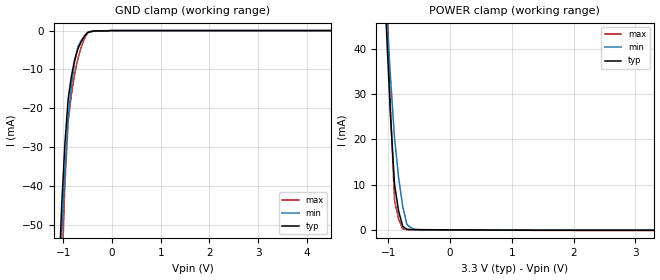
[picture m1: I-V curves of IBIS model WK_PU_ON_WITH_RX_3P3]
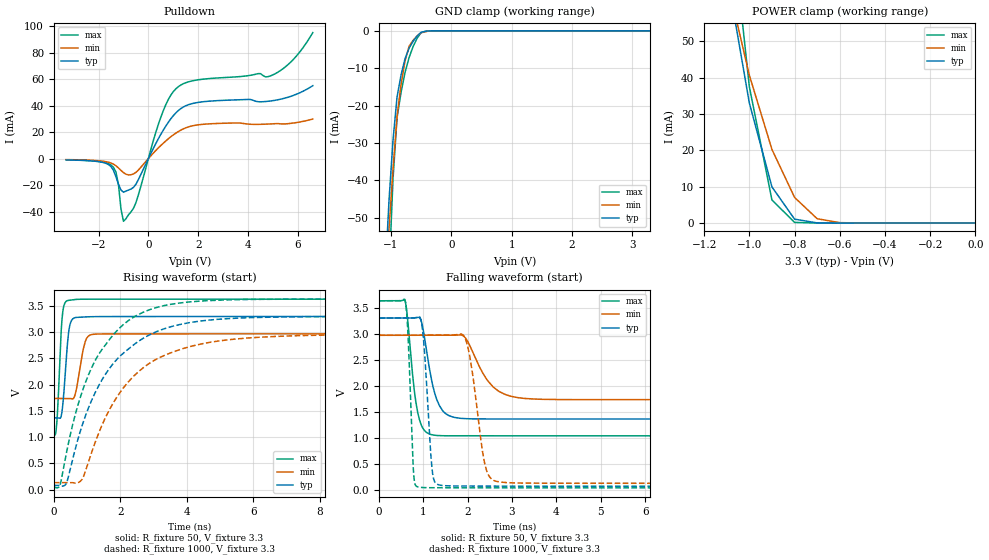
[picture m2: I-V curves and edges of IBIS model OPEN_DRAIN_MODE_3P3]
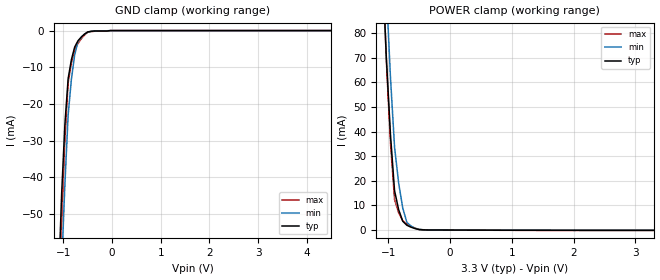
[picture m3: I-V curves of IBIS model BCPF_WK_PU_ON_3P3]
[IBIS Ver]   4.1
[File Name]   sprm821.ibs
[File Rev]   1.0
[Date]   AUG 26, 2022
[Source]   File originated at Texas Instruments
[Copyright]   (c) 2012, Texas Instruments Inc.
[Component]   f280013xpt
[Manufacturer] Texas Instruments
[Package]
| Variable   Typ   Min   Max
R_pkg   0.2934   0.1557	0.4245
L_pkg   4.2245E-09   3.1551E-09	5.6564E-09
C_pkg   0.1217E-12   0.1033E-12	0.1681E-12
[Pin]   signal_name   model_name   R_pin   L_pin   C_pin
1	GPIO29	BCF3385DSHYPBFZ_LC_IOTB_USF	0.3228	4.523E-09	0.1064E-12
2	GPIO28	BCF3385DSHYPBFZ_LC_IOTB_USF	0.2965	4.1675E-09	0.118E-12
3	XRSn	BQ0491FS_CORNER_USF	0.2785	3.9444E-09	0.1126E-12
4	GPIO228/GPIO226	BCF3385DSHYPBFZ_LC_IOTB_USF	0.2797	4.0053E-09	0.1254E-12
5	GPIO242	BCF3385DSHYPBFZ_LC_IOTB_USF	0.2922	3.9777E-09	0.1134E-12
6	GPIO224	BCF3385DSHYPBFZ_LC_IOTB_USF	0.2792	3.9066E-09	0.1072E-12
7	A15/C7/CMP1/C4/A14/ADCINCAL/CMP3P	ICF33SHYPB_LC_IOTB	0.2723	3.8915E-09	0.1178E-12
8	A11/C0/CMP1/TESTANA0	ICF33SHYPB_LC_IOTB	0.2836	3.9267E-09	0.1144E-12
9	A5/C2/CMP3	ICF33SHYPB_LC_IOTB	0.3023	4.103E-09	0.118E-12
10	A1/CMP1P	ICF33SHYPB_LC_IOTB	0.3103	4.279E-09	0.1225E-12
11	A0/C15/CMP3P/DACOUT	ICF33SHYPB_LC_IOTB	0.3335	4.5805E-09	0.1289E-12
12	VREFHIAC   NC	0.3429	4.9086E-09	0.1339E-12
13	VREFLOAC	NC	0.3405	4.9064E-09	0.1276E-12
14	A12/C1/TESTANA1/CMP2/CMP4P	ICF33SHYPB_LC_IOTB	0.338	4.6521E-09	0.1236E-12
15	A7/C3/CMP4	ICF33SHYPB_LC_IOTB	0.3031	4.2236E-09	0.1181E-12
16	A8/C11/CMP2P/CMP4P	ICF33SHYPB_LC_IOTB	0.3033	4.1416E-09	0.1184E-12
17	VSSA   NC	0.1703	3.4848E-09	0.1321E-12
18	VDDA	NC	0.17	3.5225E-09	0.1298E-12
19	A4/C14/CMP2P/CMP4	ICF33SHYPB_LC_IOTB	0.3247	4.3603E-09	0.1138E-12
20	GPIO227	BCF3385DSHYPBFZ_LC_IOTB_USF	0.3241	4.4381E-09	0.1166E-12
21	GPIO230	BCF3385DSHYPBFZ_LC_IOTB_USF	0.3443	4.676E-09	0.1242E-12
22	VSS	NC	0.2025	4.2124E-09	0.142E-12
23	GPIO13	BCF3385DSHYPBFZ_LC_IOTB_USF	0.3795	5.1624E-09	0.1315E-12
24	GPIO12	BCF3385DSHYPBFZ_LC_IOTB_USF	0.4245	5.6564E-09	0.1184E-12
25	GPIO33	BCF3385DSHYPBFZ_LC_IOTB_USF	0.3505	4.9001E-09	0.1089E-12
26	GPIO16	BCF3385DSHYPBFZ_LC_IOTB_USF	0.3121	4.3857E-09	0.119E-12
27	GPIO24	BCF3385DSHYPBFZ_LC_IOTB_USF	0.2948	4.1306E-09	0.1154E-12
28	JTAG_TCK	BCF3355DSHYPBFZ_TMS_USF	0.2795	3.9315E-09	0.1124E-12
29	GPIO37/TDO	BCPF335585DSHYPBFZ_LC_IOTB_USF	0.2792	3.8954E-09	0.11E-12
30	JTAG_TMS	BCF3355DSHYPBFZ_TMS_USF	0.285	3.9265E-09	0.1093E-12
31	GPIO35/TDI	BCF3385DSHYPBFZ_LC_IOTB_USF	0.2924	4.0293E-09	0.1117E-12
32	GPIO32	BCF3385DSHYPBFZ_LC_IOTB_USF	0.3053	4.1877E-09	0.1178E-12
33	GPIO18/X2	BCF3385DSHYPBFZ_LC_IOTB_USF	0.3239	4.4555E-09	0.1398E-12
34	GPIO19/X1/ExtR	BCPF335585DSHYPBFZ_LC_IOTB_USF	0.3322	4.691E-09	0.1598E-12
35	VDDSFL	NC	0.3546	4.8328E-09	0.1681E-12
36	VDD	NC	0.1872	4.1765E-09	0.1541E-12
37	VSS	NC	0.3525	5.0672E-09	0.1332E-12
38	GPIO4	BCF3385DSHYPBFZ_LC_IOTB_USF	0.3129	4.3589E-09	0.1183E-12
39	GPIO3	BCF3385DSHYPBFZ_LC_IOTB_USF	0.2952	4.1162E-09	0.1162E-12
40	GPIO2	BCF3385DSHYPBFZ_LC_IOTB_USF	0.2811	3.9281E-09	0.1137E-12
41	GPIO1	BCF3385DSHYPBFZ_LC_IOTB_USF	0.273	3.7821E-09	0.1112E-12
42	GPIO0	BCF3385DSHYPBFZ_LC_IOTB_USF	0.2691	3.7414E-09	0.1053E-12
43	GPIO7	BCF3385DSHYPBFZ_LC_IOTB_USF	0.2701	3.717E-09	0.1058E-12
44	VSS	NC	0.1557	3.1742E-09	0.125E-12
45	VDD	NC	0.156	3.1551E-09	0.1294E-12
46	VDDSFL	NC	0.2897	4.0015E-09	0.1177E-12
47	GPIO5	BCF3385DSHYPBFZ_LC_IOTB_USF	0.3004	4.1883E-09	0.1193E-12
48	GPIO6	BCF3385DSHYPBFZ_LC_IOTB_USF	0.311	4.353E-09	0.1033E-12
| End of package information
|   Component BQ0491FS_CORNER_USF
[Component]   BQ0491FS_CORNER_USF
[Manufacturer]   Texas Instruments
[Package]
|  variable   typ   min   max
R_pkg   0   0   0
L_pkg   0   0   0
C_pkg   0   0   0
[Pin]   signal_name   model_name   R_pin   L_pin   C_pin
VSS   VSS   GND
VDDS   VDDS   POWER
PAD   PAD   BQ0491FS_CORNER_USF
[Model Selector] BQ0491FS_CORNER_USF
WK_PU_ON_WITH_RX_3P3  Cell operated at 3.3(nom)
|WK_PU_ON_WITH_RX_3P3; WEAK_PULLUP_ON_WITH_RX
OPEN_DRAIN_MODE_3P3  Cell operated at 3.3(nom)
|   Component BCPF335585DSHYPBFZ_LC_IOTB_USF
[Component]   BCPF335585DSHYPBFZ_LC_IOTB_USF
[Manufacturer]   Texas Instruments
[Package]
|  variable   typ   min   max
R_pkg   0   0   0
L_pkg   0   0   0
C_pkg   0   0   0
[Pin]   signal_name   model_name   R_pin   L_pin   C_pin
VSS   VSS   GND
VDDS   VDDS   POWER
PAD   PAD   BCPF335585DSHYPBFZ_LC_IOTB_USF
[Model Selector] BCPF335585DSHYPBFZ_LC_IOTB_USF
BCPF_WK_PU_ON_3P3  Cell operated at 3.3(nom)
|BCPF_WK_PU_ON_3P3; WEAK_PULLUP_ON
BCPF_DRIVER_MODE_4MA_3P3  Cell operated at 3.3(nom)
|BCPF_DRIVER_MODE_4MA_3P3
BCPF_DRIVER_MODE_2MA_3P3  Cell operated at 3.3(nom)
|BCPF_DRIVER_MODE_2MA_3P3
BCPF_WK_PD_ON_3P3  Cell operated at 3.3(nom)
|   Component ICF33SHYPB_LC_IOTB
[Component]   ICF33SHYPB_LC_IOTB
[Manufacturer]   Texas Instruments
[Package]
|  variable   typ   min   max
R_pkg   0   0   0
L_pkg   0   0   0
C_pkg   0   0   0
[Pin]   signal_name   model_name   R_pin   L_pin   C_pin
VSS   VSS   GND
VDDS   VDDS   POWER
PAD   PAD   ICF33SHYPB_LC_IOTB
[Model Selector] ICF33SHYPB_LC_IOTB
ICF_RECEIVER_MODE_3P3  Cell operated at 3.3(nom)
|ICF_RECEIVER_MODE_3P3; RECEIVER_MODE
ICF_WK_PU_ON_3P3  Cell operated at 3.3(nom)
|ICF_WK_PU_ON_3P3; WEAK_PULLUP_ON
ICF_WK_PD_ON_3P3  Cell operated at 3.3(nom)
|   Component BCF3385DSHYPBFZ_LC_IOTB_USF
[Component]   BCF3385DSHYPBFZ_LC_IOTB_USF
[Manufacturer]   Texas Instruments
[Package]
|  variable   typ   min   max
R_pkg   0   0   0
L_pkg   0   0   0
C_pkg   0   0   0
[Pin]   signal_name   model_name   R_pin   L_pin   C_pin
VSS   VSS   GND
VDDS   VDDS   POWER
PAD   PAD   BCF3385DSHYPBFZ_LC_IOTB_USF
[Model Selector] BCF3385DSHYPBFZ_LC_IOTB_USF
BCF_WK_PU_ON_3P3  Cell operated at 3.3(nom)
|BCF_WK_PU_ON_3P3; WEAK_PULLUP_ON
BCF_WK_PD_ON_3P3  Cell operated at 3.3(nom)
|BCF_WK_PD_ON_3P3; WEAK_PULLDOWN_ON
BCF_DRIVER_MODE_3P3  Cell operated at 3.3(nom)
|BCF_DRIVER_MODE_3P3
BCF_RECEIVER_MODE_3P3  Cell operated at 3.3(nom)
|   Component BCF3355DSHYPBFZ_TMS_USF
[Component]   BCF3355DSHYPBFZ_TMS_USF
[Manufacturer]   Texas Instruments
[Package]
|  variable   typ   min   max
R_pkg   0   0   0
L_pkg   0   0   0
C_pkg   0   0   0
[Pin]   signal_name   model_name   R_pin   L_pin   C_pin
VSS   VSS   GND
VDDS   VDDS   POWER
PAD   PAD   BCF3355DSHYPBFZ_TMS_USF
[Model Selector] BCF3355DSHYPBFZ_TMS_USF
TMS_WK_PU_ON_3P3  Cell operated at 3.3(nom)
|TMS_WK_PU_ON_3P3; WEAK_PULLUP_ON
TMS_DRIVER_3P3  Cell operated at 3.3(nom)
|TMS_DRIVER_3P3
TMS_WK_PD_ON_3P3  Cell operated at 3.3(nom)
| Models and submodels in the file (16): WK_PU_ON_WITH_RX_3P3 (Input), OPEN_DRAIN_MODE_3P3 (I/O_open_drain), BCPF_WK_PU_ON_3P3 (Input), BCPF_DRIVER_MODE_4MA_3P3 (I/O), BCPF_DRIVER_MODE_2MA_3P3 (I/O), BCPF_WK_PD_ON_3P3 (Input), ICF_RECEIVER_MODE_3P3 (Input), ICF_WK_PU_ON_3P3 (Input), ICF_WK_PD_ON_3P3 (Input), BCF_WK_PU_ON_3P3 (Input), BCF_WK_PD_ON_3P3 (Input), BCF_DRIVER_MODE_3P3 (I/O), BCF_RECEIVER_MODE_3P3 (Input), TMS_WK_PU_ON_3P3 (Input), TMS_DRIVER_3P3 (I/O), TMS_WK_PD_ON_3P3 (Input)
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|OPEN_DRAIN_MODE_3P3
|   Model Cell WK_PU_ON_WITH_RX_3P3
|WK_PU_ON_WITH_RX_3P3
[Model]   WK_PU_ON_WITH_RX_3P3
Model_type   Input
Polarity   Non-Inverting
Vinl =  0.8
Vinh =  2
C_comp   1.11773p   1.013376p   1.244487p
[Model Spec]
Vinl   0.8   0.8   0.8
Vinh   2   2   2
[Temperature Range]   25   155   -40
[Voltage Range]   3.3   2.97   3.63
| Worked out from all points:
|   GND clamp passes 1 mA (typ) near -0.54 V on its own axis
|   POWER clamp passes 1 mA (typ) near -0.77 V on its own axis
| Nom Voltages:
|   BIASFET=3.3, VDD=1.2, VDDS=3.3, VSS=0
| Min Voltages:
|   BIASFET=2.97, VDD=1.08, VDDS=2.97, VSS=0
| Max Voltages:
|   BIASFET=3.63, VDD=1.32, VDDS=3.63, VSS=0
[POWER_clamp]
|   voltage   I(typ)   I(min)   I(max)
-3.3V     1.132A     1.059A     1.769A
-1.033V   45.08mA    49.59mA    56.93mA
-966.7mV  25.39mA    33.9mA     27.23mA
-900mV    10.01mA    20.29mA    6.454mA
-833.3mV  4.092mA    11.48mA    2.326mA
-766.7mV  785.4uA    5.125mA    201.1uA
-700mV    89.29uA    1.212mA    78.7uA
-633.3mV  61.2uA     494uA      69.62uA
-566.7mV  44.07uA    99.73uA    61.24uA
3.3V      -85.93uA   -55.95uA   -137.9uA
[GND_clamp]
|   voltage   I(typ)   I(min)   I(max)
-3.3V     -1.198A    -966mA     -2.548A
-1.1V     -66.27mA   -70.87mA   -99.83mA
-1.033V   -45.41mA   -52.93mA   -65.12mA
-966.7mV  -29.23mA   -36.93mA   -39.6mA
-900mV    -17.72mA   -22.86mA   -23.27mA
-833.3mV  -11.83mA   -14.27mA   -16.55mA
-766.7mV  -7.493mA   -8.038mA   -11.21mA
-700mV    -4.704mA   -4.168mA   -7.263mA
-566.7mV  -1.465mA   -1.376mA   -2.095mA
-500mV    -469.8uA   -575.8uA   -591.3uA
-33.33mV  0A         0A         0A
6.6V      0A         0A         0A
|   Model Cell OPEN_DRAIN_MODE_3P3
|OPEN_DRAIN_MODE_3P3
[Model]   OPEN_DRAIN_MODE_3P3
Model_type   I/O_open_drain
Polarity   Non-Inverting
Enable   Active-Low
Vinl =  0.8
Vinh =  2
Cref =  15.0000pF
Rref =  100.0000M
Vref =  0V
Vmeas =  1.65
C_comp   1.11773p   1.013376p   1.244487p
[Model Spec]
Vinl   0.8   0.8   0.8
Vinh   2   2   2
[Temperature Range]   25   155   -40
[Voltage Range]   3.3   2.97   3.63
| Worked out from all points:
|   slope of the pulldown table from 0 to 0.495 V, typ, clamps not added: 27.3 ohm
|   GND clamp passes 1 mA (typ) near -0.54 V on its own axis
|   POWER clamp passes 1 mA (typ) near -0.79 V on its own axis
|   rising waveform, R_fixture 50, V_fixture 3.3: 20-80 % time 139ps typ, 204ps min, 112ps max; typ from 1.37 V to 3.3 V
|   rising waveform, R_fixture 1000, V_fixture 3.3: 20-80 % time 1.57ns typ, 1.73ns min, 1.34ns max; typ from 0.081 V to 3.3 V
|   falling waveform, R_fixture 50, V_fixture 3.3: 20-80 % time 266ps typ, 495ps min, 195ps max; typ from 3.3 V to 1.37 V
|   falling waveform, R_fixture 1000, V_fixture 3.3: 20-80 % time 138ps typ, 264ps min, 97ps max; typ from 3.3 V to 0.081 V
| Nom Voltages:
|   BIASFET=3.3, VDD=1.2, VDDS=3.3, VSS=0
| Min Voltages:
|   BIASFET=2.97, VDD=1.08, VDDS=2.97, VSS=0
| Max Voltages:
|   BIASFET=3.63, VDD=1.32, VDDS=3.63, VSS=0
[POWER_clamp]
|   voltage   I(typ)   I(min)   I(max)
-3.3V     1.132A     1.059A     1.769A
-1.067V   57.04mA    58.46mA    76.19mA
-1.033V   45.04mA    49.58mA    56.86mA
-1V       33.04mA    40.7mA     37.54mA
-900mV    9.95mA     20.27mA    6.36mA
-800mV    1.073mA    7.058mA    176.5uA
-700mV    35.88uA    1.186mA    3.424uA
-600mV    1.374uA    110.7uA    455.3nA
0V        338.2pA    5.96nA     285.2pA
[Pulldown]
|   voltage   I(typ)   I(min)   I(max)
-3.3V     -1.018mA   -784.1uA   -895.6uA
-1.4V     -8.945mA   -4.198mA   -6.606mA
-1.2V     -19.44mA   -7.097mA   -19.74mA
-1.1V     -23.79mA   -8.926mA   -38.1mA
-1V       -25.42mA   -10.61mA   -47.4mA
-500mV    -19.36mA   -10.45mA   -33.38mA
500mV     18.33mA    9.885mA    31.3mA
1.1V      34.47mA    19.21mA    52.67mA
2.1V      42.73mA    25.73mA    59.79mA
4.9V      43.52mA    26.17mA    62.49mA
5.8V      47.6mA     26.81mA    74.57mA
6.6V      55.08mA    29.87mA    95.23mA
[GND_clamp]
|   voltage   I(typ)   I(min)   I(max)
-3.3V     -1.198A    -966mA     -2.548A
-1.1V     -66.26mA   -70.86mA   -99.82mA
-1.033V   -45.39mA   -52.93mA   -65.1mA
-966.7mV  -29.21mA   -36.92mA   -39.58mA
-900mV    -17.69mA   -22.85mA   -23.24mA
-833.3mV  -11.79mA   -14.25mA   -16.46mA
-766.7mV  -7.428mA   -8.019mA   -11.09mA
-700mV    -4.622mA   -4.142mA   -7.129mA
-566.7mV  -1.379mA   -1.338mA   -1.958mA
-500mV    -383.7uA   -535.9uA   -452.8uA
-300mV    -821.5nA   -7.147uA   -404.1nA
3.3V      338.2pA    143.1nA    239.5pA
[Ramp]
| variable   typ   min   max
dV/dt_f  1.1674782/0.26758435n 0.74431688/0.49748067n  1.5612158/0.19548637n
dV/dt_r 16.566269m/0.16851048n 10.821448m/0.18717204n 21.089911m/0.14213015n
R_load = 50
[Rising Waveform]
R_fixture = 50
V_fixture = 3.3
V_fixture_min = 2.97
V_fixture_max = 3.63
|   time   V(typ)   V(min)   V(max)
0s        1.368V     1.738V     1.045V
85.1ps    1.368V     1.738V     1.237V
222.8ps   1.404V     1.738V     3.038V
302.4ps   1.849V     1.738V     3.503V
480.8ps   3.134V     1.739V     3.611V
650.9ps   3.28V      1.835V     3.625V
883.3ps   3.29V      2.667V     3.629V
1.085ns   3.296V     2.946V     3.63V
2.138ns   3.3V       2.969V     3.63V
500ns     3.3V       2.97V      3.63V
[Rising Waveform]
R_fixture = 1000
V_fixture = 3.3
V_fixture_min = 2.97
V_fixture_max = 3.63
|   time   V(typ)   V(min)   V(max)
0s        81.2mV     135.1mV    50.52mV
192.5ps   77.67mV    135.1mV    97.37mV
387.1ps   134.1mV    135mV      724.8mV
838.5ps   1.197V     186.7mV    1.84V
1.379ns   2.014V     1.122V     2.607V
1.98ns    2.537V     1.841V     3.081V
2.544ns   2.825V     2.247V     3.337V
3.332ns   3.068V     2.56V      3.51V
5.837ns   3.277V     2.89V      3.625V
500ns     3.3V       2.97V      3.63V
[Falling Waveform]
R_fixture = 50
V_fixture = 3.3
V_fixture_min = 2.97
V_fixture_max = 3.63
|   time   V(typ)   V(min)   V(max)
0s        3.3V       2.97V      3.63V
583ps     3.3V       2.97V      3.638V
803.8ps   3.302V     2.97V      1.863V
915.1ps   3.309V     2.97V      1.349V
1.254ns   1.867V     2.97V      1.057V
1.503ns   1.472V     2.97V      1.047V
1.948ns   1.375V     2.922V     1.047V
2.701ns   1.368V     1.897V     1.046V
4.266ns   1.368V     1.739V     1.045V
500ns     1.368V     1.738V     1.045V
[Falling Waveform]
R_fixture = 1000
V_fixture = 3.3
V_fixture_min = 2.97
V_fixture_max = 3.63
|   time   V(typ)   V(min)   V(max)
0s        3.3V       2.97V      3.63V
597.9ps   3.3V       2.97V      3.609V
783.5ps   3.301V     2.97V      294.5mV
944.1ps   3.272V     2.97V      59.09mV
1.149ns   937.5mV    2.97V      52.6mV
1.266ns   149.7mV    2.97V      52.01mV
1.948ns   84.58mV    2.907V     50.29mV
2.499ns   83.13mV    253.5mV    50.07mV
3.393ns   81.49mV    140.3mV    50.06mV
500ns     81.2mV     135.1mV    50.06mV
|BCPF_WK_PD_ON_3P3; WEAK_PULLDOWN_ON
|   Model Cell BCPF_WK_PU_ON_3P3
|BCPF_WK_PU_ON_3P3
[Model]   BCPF_WK_PU_ON_3P3
Model_type   Input
Polarity   Non-Inverting
Vinl =  0.8
Vinh =  2
C_comp   1.21982p   0.982413p   1.3757p
[Model Spec]
Vinl   0.8   0.8   0.8
Vinh   2   2   2
[Temperature Range]   25   155   -40
[Voltage Range]   3.3   2.97   3.63
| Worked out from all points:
|   GND clamp passes 1 mA (typ) near -0.57 V on its own axis
|   POWER clamp passes 1 mA (typ) near -0.61 V on its own axis
| Nom Voltages:
|   BIASFET=3.3, VDD=1.2, VDDS=3.3, VSS=0
| Min Voltages:
|   BIASFET=2.97, VDD=1.08, VDDS=2.97, VSS=0
| Max Voltages:
|   BIASFET=3.63, VDD=1.32, VDDS=3.63, VSS=0
[POWER_clamp]
|   voltage   I(typ)   I(min)   I(max)
-3.3V     1.919A     2.431A     2.069A
-1.1V     109.8mA    140.8mA    113.2mA
-1.033V   70.21mA    98.04mA    69.24mA
-966.7mV  38.95mA    62.35mA    35.63mA
-900mV    16.03mA    33.73mA    12.36mA
-833.3mV  8.266mA    19.09mA    7.029mA
-766.7mV  3.571mA    8.879mA    3.722mA
-700mV    1.939mA    3.079mA    2.444mA
-566.7mV  603.9uA    711.2uA    759.2uA
-500mV    195.8uA    269.7uA    227.2uA
-366.7mV  40.85uA    44.56uA    53.2uA
3.3V      -108.8uA   -62.99uA   -174uA
[GND_clamp]
|   voltage   I(typ)   I(min)   I(max)
-3.3V     -1.48A     -1.41A     -2.182A
-1.1V     -69.91mA   -89.89mA   -82.68mA
-1.033V   -44.46mA   -64.18mA   -52.64mA
-966.7mV  -25.52mA   -41.89mA   -29.83mA
-900mV    -13.08mA   -23mA      -14.24mA
-833.3mV  -7.945mA   -13.29mA   -8.83mA
-766.7mV  -4.523mA   -6.66mA    -5.269mA
-700mV    -2.817mA   -3.105mA   -3.556mA
-566.7mV  -980.5uA   -1.002mA   -1.249mA
-500mV    -376.2uA   -438.1uA   -476.5uA
-33.33mV  0A         0A         0A
6.6V      0A         0A         0A
